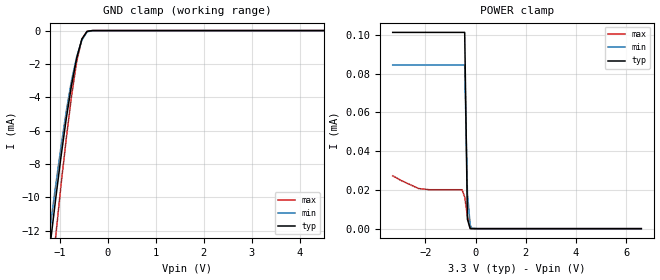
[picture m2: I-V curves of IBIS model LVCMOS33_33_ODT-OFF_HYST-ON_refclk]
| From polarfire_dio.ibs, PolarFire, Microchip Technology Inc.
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|   Model LVCMOS33_33_ODT-OFF_HYST-ON_refclk
[Model]   LVCMOS33_33_ODT-OFF_HYST-ON_refclk
Model_type   Input
Vinl =   0.8
Vinh =   2.0
|   typ   min   max
C_comp   5.210e-12   5.210e-12   5.520e-12
[Temperature Range]  25C   100C   -40C
[Voltage Range]  3.3   3.135   3.465
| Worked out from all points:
|   GND clamp passes 1 mA (typ) near -0.59 V on its own axis
[GND Clamp]
| Voltage   I(typ)   I(min)   I(max)
-3.3V     -81.73mA   -75.27mA   -93.52mA
-1.408V   -18.01mA   -16.5mA    -21.72mA
-1.191V   -12.56mA   -11.55mA   -15.38mA
-1.083V   -9.973mA   -9.186mA   -12.23mA
-974.5mV  -7.519mA   -6.929mA   -9.214mA
-866.2mV  -5.259mA   -4.836mA   -6.455mA
-758mV    -3.292mA   -3.006mA   -3.951mA
-649.7mV  -1.65mA    -1.574mA   -1.856mA
-541.4mV  -510.1uA   -568.4uA   -505.8uA
-433.1mV  -46.69uA   -75.87uA   -45.55uA
-108.3mV  11nA       -4.164nA   -4.033nA
6.6V      0A         0A         0A
[POWER Clamp]
| Voltage   I(typ)   I(min)   I(max)
-3.3V     101.3uA    84.44uA    27.25uA
-2.274V   101.3uA    84.44uA    20.72uA
-1.841V   101.3uA    84.44uA    20.09uA
-541.4mV  101.3uA    84.44uA    20.09uA
-433.1mV  101.3uA    84.44uA    16.37uA
-324.8mV  4.863uA    18.34uA    6.484uA
-216.6mV  91.72nA    2.076uA    85.37nA
-165mV    12.82nA    167.8nA    73.68nA
103.1mV   0A         0A         0A
6.6V      0A         0A         0A
